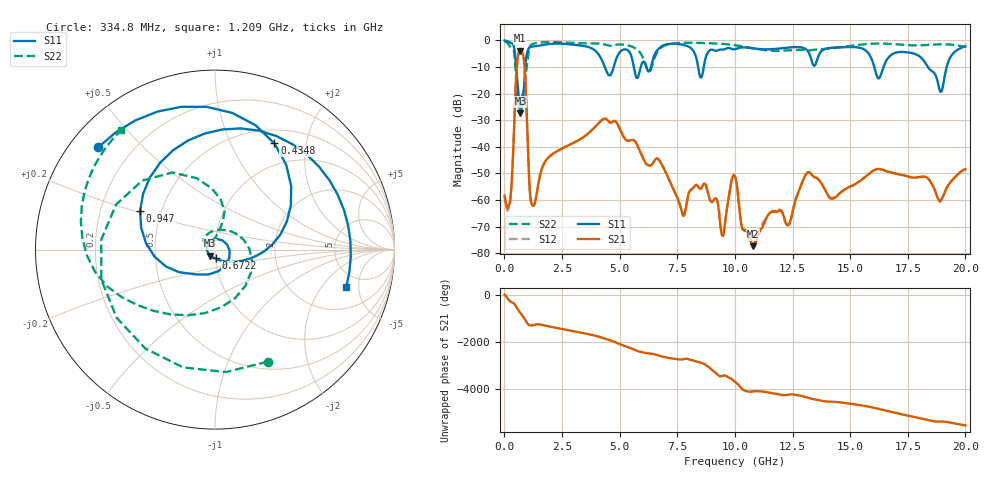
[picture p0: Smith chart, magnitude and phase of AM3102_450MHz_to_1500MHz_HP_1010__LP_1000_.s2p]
!Agilent Technologies,E8364B,MY43040894,A.07.50.67
!Agilent E8364B: A.07.50.67
!Date: Thursday, January 11, 2018 06:12:14
!Correction: S11(Full 2 Port(1,2))
!S21(Full 2 Port(1,2))
!S12(Full 2 Port(1,2))
!S22(Full 2 Port(1,2))
!S2P File: Measurements: S11, S21, S12, S22:
# Hz S  dB  R 50
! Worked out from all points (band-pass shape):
!   1601 points, 10 MHz to 20 GHz, reference 50 ohm
!   highest |S21| = -3.90 dB at 684.7 MHz (marker M1); lowest = -77.4 dB at 10.79 GHz (marker M2)
!   |S21| within 3 dB of the highest: 573.2 MHz to 842.6 MHz (269.4 MHz wide, 38.1 % of centre)
!   lowest |S11| = -27.4 dB at 697.2 MHz (marker M3), VSWR 1.09, Z = 47.4 - j3.21 ohm
!   |S11| at or under -10 dB: 510.8 MHz to 904 MHz (393.2 MHz wide, 55.6 % of centre); 16.05 GHz to 16.45 GHz (401.2 MHz wide, 2.47 % of centre); 18.37 GHz to 19.19 GHz (816.5 MHz wide, 4.35 % of centre)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
!   |S22| runs from -26.3 to -0.4 dB; largest |S21 - S12| = 0.00063
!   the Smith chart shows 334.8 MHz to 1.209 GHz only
!   S11 on the Smith chart (normalised r, x): 334.8 MHz: 0.08, +0.37; 434.8 MHz: 0.68, +1.48; 672.2 MHz: 1.00, -0.10; 947 MHz: 0.38, +0.21; 1.209 GHz: 3.61, -3.60
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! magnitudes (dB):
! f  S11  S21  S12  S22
! 10 MHz  -0.1  -58.7  -57.7  -0.4
! 334.8 MHz  -1.3  -50.7  -51.0  -3.2
! 434.8 MHz  -3.4  -29.4  -29.4  -5.1
! 672.2 MHz  -26.2  -3.9  -3.9  -25.9
! 684.7 MHz  -27.1  -3.9  -3.9  -25.4
! 697.2 MHz  -27.4  -3.9  -3.9  -24.8
! 947 MHz  -6.6  -22.7  -22.7  -11.6
! 1.209 GHz  -2.4  -61.9  -61.8  -1.4
! 1.834 GHz  -1.5  -44.8  -44.9  -0.7
! 3.346 GHz  -2.0  -36.9  -36.9  -1.1
! 5.757 GHz  -14.2  -39.2  -39.2  -3.5
! 6.682 GHz  -3.3  -44.7  -44.7  -3.8
! 7.756 GHz  -1.7  -65.9  -65.2  -1.0
! 8.706 GHz  -7.5  -54.0  -54.0  -1.0
! 9.455 GHz  -3.5  -73.5  -73.3  -1.4
! 10.01 GHz  -3.4  -51.2  -51.2  -1.9
! 10.79 GHz  -3.0  -77.4  -76.6  -3.0
! 13.34 GHz  -8.0  -50.6  -50.7  -3.7
! 14.23 GHz  -2.8  -59.4  -59.3  -3.0
! 16.68 GHz  -6.4  -49.4  -49.5  -1.3
! 18.94 GHz  -19.4  -60.2  -60.4  -1.5
! 20 GHz  -2.3  -48.5  -48.3  -2.4
